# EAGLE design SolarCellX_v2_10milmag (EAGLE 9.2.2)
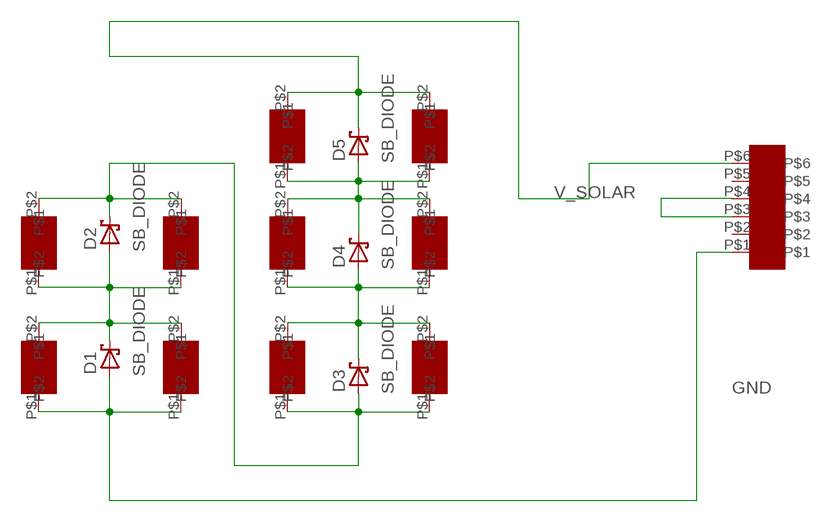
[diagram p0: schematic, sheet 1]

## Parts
1  SLMD121H04L  [SLMD121H04L]
2  SLMD121H04L  [SLMD121H04L]
11  SLMD121H04L  [SLMD121H04L]
12  SLMD121H04L  [SLMD121H04L]
13  SLMD121H04L  [SLMD121H04L]
14  SLMD121H04L  [SLMD121H04L]
21  SLMD121H04L  [SLMD121H04L]
22  SLMD121H04L  [SLMD121H04L]
23  SLMD121H04L  [SLMD121H04L]
24  SLMD121H04L  [SLMD121H04L]
D1  SB_DIODE  [SB_DIODE]
D2  SB_DIODE  [SB_DIODE]
D3  SB_DIODE  [SB_DIODE]
D4  SB_DIODE  [SB_DIODE]
D5  SB_DIODE  [SB_DIODE]
U$1  M20-8760342  [M20-8760342]

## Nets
GND: 11.P$1 12.P$1 D1.POS U$1.P$1
N$2: 11.P$2 12.P$2 13.P$1 14.P$1 D1.NEG D2.POS
N$3: 13.P$2 14.P$2 21.P$1 22.P$1 D2.NEG D3.POS
N$4: 1.P$1 2.P$1 23.P$2 24.P$2 D4.NEG D5.POS
N$5: 21.P$2 22.P$2 23.P$1 24.P$1 D3.NEG D4.POS
N$6: U$1.P$3 U$1.P$4
V_SOLAR: 1.P$2 2.P$2 D5.NEG U$1.P$6
Unconnected: U$1.P$2 U$1.P$5

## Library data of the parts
1 2 11-14 21-24 = Solar:SLMD121H04L
D1-D5 = Solar:SB_DIODE
U$1 = Solar:M20-8760342

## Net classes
1 power: width 0.254 mm

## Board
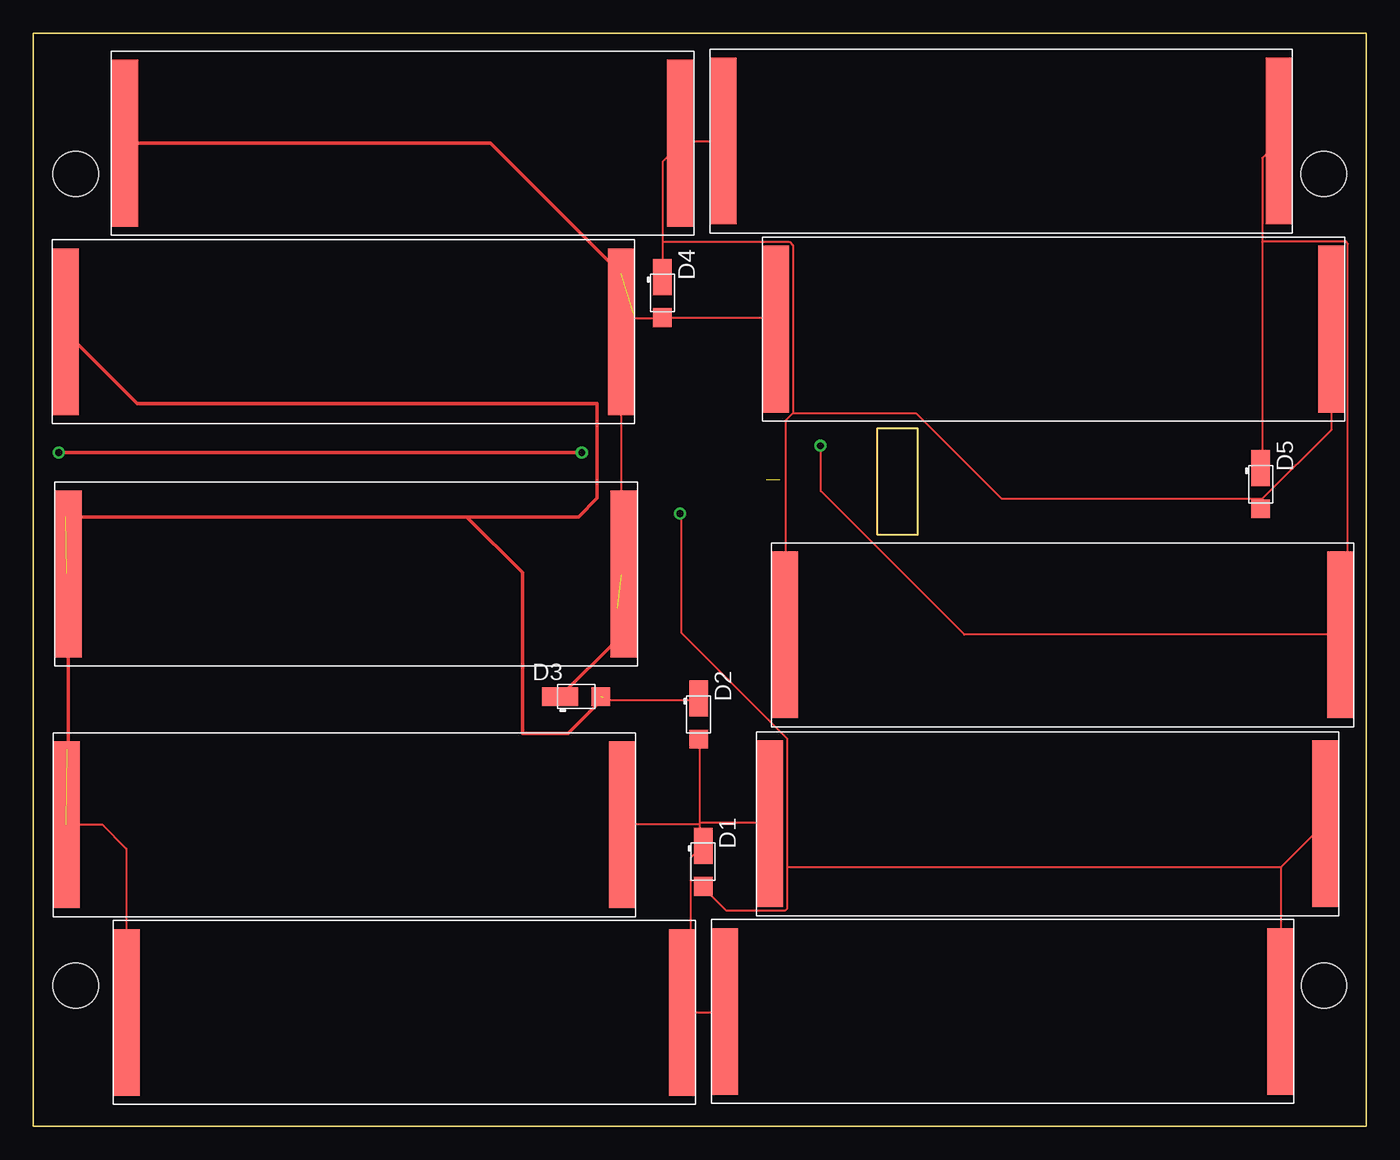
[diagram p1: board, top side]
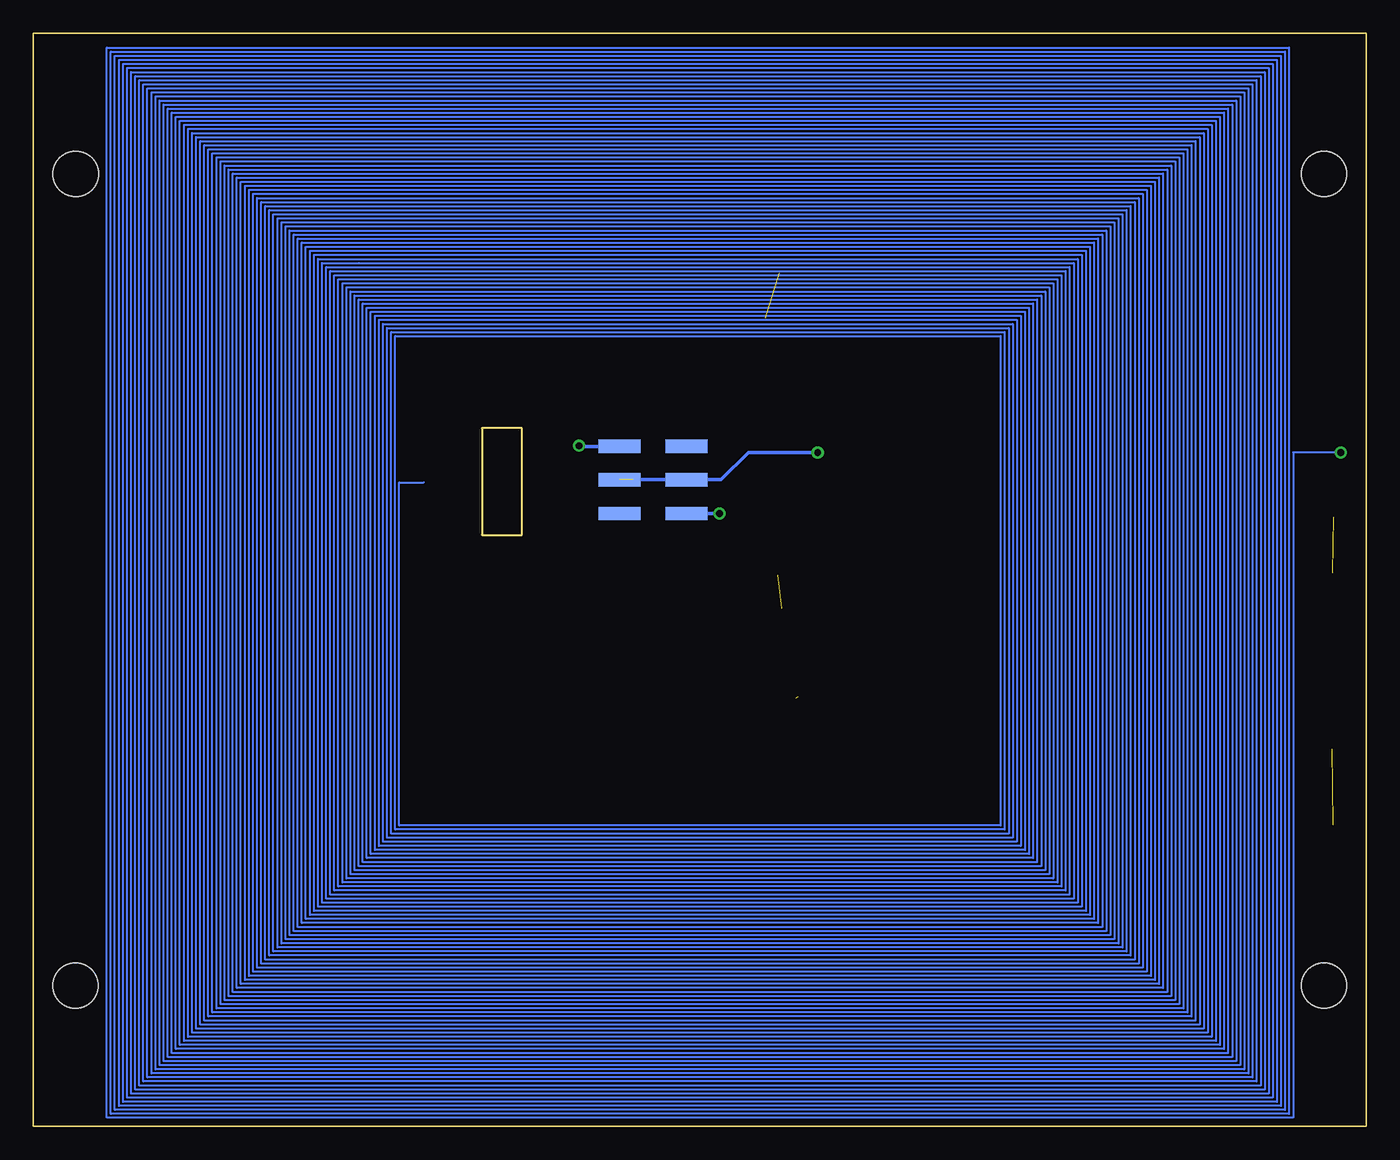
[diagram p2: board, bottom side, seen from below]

Size 100 x 82 mm. Coordinates in mm from the lower left corner, seen from the top.
Outline: 0,0 0,82 100,82 100,0 0,0
Outline: 63.35,52.37 66.35,52.37 66.35,44.37 63.35,44.37 63.35,52.37
Copper layers ([2:1+2*15+16:15]): Top 0.035559375mm / dielectric 0.17018125mm / Route2 0.01778125mm / dielectric 47mil / Route15 0.01778125mm / dielectric 0.17018125mm / Bottom 0.035559375mm
Design rules "default *": minimum track width 6mil, minimum drill 0.35mm, track to track 5mil, track to pad 6mil, pad to pad 6mil, via to via 6mil, smd to smd 6mil, copper to edge 20mil, drill to drill 6mil, minimum pad ring 10mil, minimum via ring 8mil, stop-mask expansion 4mil, vias tented up to drill 0mil, thermal gap 10mil
Holes 3.4 mm at 3.17,10.55 96.82,71.45 3.17,71.45 96.83,10.55

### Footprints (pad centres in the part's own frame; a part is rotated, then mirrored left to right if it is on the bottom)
SLMD121H04L = smd 2 x 12.5: P$1 1,6.9; P$2 42.7,6.9
SB_DIODE = smd 2.7 x 1.4: NEG -1.2,0 | smd 1.4 x 1.4: POS 1.85,0
M20-8760342 = smd 1 x 3.15: P$1 0.5,1.575; P$2 0.5,6.625; P$3 3.04,1.575; P$4 3.04,6.625; P$5 5.54,1.575; P$6 5.54,6.625

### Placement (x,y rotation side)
1  50.77,67.02 0 top
2  55.37,29.97 0 top
11  94.58,15.51 180 top
12  97.95,29.59 180 top
13  49.69,15.44 180 top
14  45.18,29.52 180 top
21  1.61,34.53 0 top
22  1.41,52.7 0 top
23  5.85,66.86 0 top
24  54.7,52.9 0 top
D1  50.26,19.85 270 top
D2  49.92,30.9 270 top
D3  40.73,32.23 0 top
D4  47.19,62.52 270 top
D5  92.08,48.17 270 top
U$1  49.4,45.47 90 bottom

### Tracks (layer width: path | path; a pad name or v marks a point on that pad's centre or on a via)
GND  (via drill 0.5)
  Top 0.152: 56.58,19.42 56.58,16.34 56.44,16.2 51.97,16.2 50.29,17.88 D1.POS | 56.58,19.42 56.58,29.06 48.62,37.02 48.62,45.96 v48.51,45.97 | 93.6,19.42 93.6,8.66 11.P$1 | 93.6,19.42 96.81,22.63 12.P$1 | 93.6,19.42 56.58,19.42
  Bottom 0.254: U$1.P$1 v48.51,45.97
N$2
  Top 0.152: 49.31,8.52 51.83,8.52 11.P$2 | 49.31,8.52 48.76,8.52 13.P$1 49.31,8.52 | 50.01,22.63 50.01,21.23 50.15,21.09 D1.NEG 50.15,20.95 49.31,20.12 49.31,8.52 | 50.01,22.63 50.01,22.77 | 50.01,22.77 50.01,28.92 D2.POS | 50.01,22.77 55.18,22.77 12.P$2 | 50.01,22.63 44.28,22.63 14.P$1
N$3  (3 unrouted)
  Top 0.152: 14.P$2 2.52,22.63 5.17,22.63 6.99,20.82 6.99,8.66 13.P$2 | D2.NEG 49.87,31.99 42.49,31.99 D3.POS | 2.52,59.51 22.P$1 | 2.52,41.49 21.P$1
  Top 0.254: 22.P$1 7.78,54.23 42.29,54.23 42.29,47.12 40.89,45.72 32.51,45.72 | 32.51,45.72 2.41,45.72 | 21.P$1 2.61,28.39 2.54,28.32 | 32.51,45.72 36.7,41.53 36.7,29.46 40.13,29.46 42.8,32.13
N$4
  Top 0.152: 92.2,47.08 92.2,46.38 D5.POS | 92.2,47.08 97.37,52.25 97.37,59.79 24.P$2 | 47.22,66.36 47.22,72.36 48.48,73.62 23.P$2 48.62,73.76 48.76,73.9 51.69,73.9 1.P$1 | 47.22,66.36 47.22,63.84 D4.NEG | 57,53.51 56.44,52.95 56.44,36.88 2.P$1 | 57,53.51 57,66.08 56.72,66.36 47.22,66.36 | 92.2,47.08 72.64,47.08 66.22,53.51 57,53.51
N$5  (2 unrouted)
  Top 0.152: 24.P$1 55.6,59.93 54.9,60.63 47.22,60.63 D4.POS 47.08,60.63 45.12,60.63 44.15,59.65 22.P$2 44.15,59.51 44.15,41.35 | 44.15,41.35 44.28,41.35 21.P$2 44.15,41.35 | 6.99,73.62 23.P$1
  Top 0.254: 23.P$1 34.32,73.76 44.07,64.01 | D3.NEG 43.81,36.52 43.81,38.86
N$6  (via drill 0.5)  (1 unrouted)
  Top 0.254: v41.15,50.55 v1.91,50.55
  Bottom 0.152: v1.91,50.55 5.49,50.55 5.49,0.65 94.49,0.65 94.49,80.92 5.79,80.92 5.79,0.91 94.18,0.91 94.18,80.62 6.1,80.62 6.1,1.22 93.88,1.22 93.88,80.31 6.4,80.31 6.4,1.52 93.57,1.52 93.57,80.01 6.71,80.01 6.71,1.83 93.27,1.83 93.27,79.7 7.01,79.7 7.01,2.13 92.96,2.13 92.96,79.4 7.32,79.4 7.32,2.44 92.66,2.44 92.66,79.1 7.62,79.1 7.62,2.74 92.35,2.74 92.35,78.79 7.92,78.79 7.92,3.05 92.05,3.05 92.05,78.49 8.23,78.49 8.23,3.35 91.75,3.35 91.75,78.18 8.53,78.18 8.53,3.66 91.44,3.66 91.44,77.88 8.84,77.88 8.84,3.96 91.14,3.96 91.14,77.57 9.14,77.57 9.14,4.27 90.83,4.27 90.83,77.27 9.45,77.27 9.45,4.57 90.53,4.57 90.53,76.96 9.75,76.96 9.75,4.88 90.22,4.88 90.22,76.66 10.06,76.66 10.06,5.18 89.92,5.18 89.92,76.35 10.36,76.35 10.36,5.49 89.61,5.49 89.61,76.05 10.67,76.05 10.67,5.79 89.31,5.79 89.31,75.74 10.97,75.74 10.97,6.1 89,6.1 89,75.44 11.28,75.44 11.28,6.4 88.7,6.4 88.7,75.13 11.58,75.13 11.58,6.71 88.39,6.71 88.39,74.83 11.89,74.83 11.89,7.01 88.09,7.01 88.09,74.52 12.19,74.52 12.19,7.32 87.78,7.32 87.78,74.22 12.5,74.22 12.5,7.62 87.48,7.62 87.48,73.91 12.8,73.91 12.8,7.92 87.17,7.92 87.17,73.61 13.11,73.61 13.11,8.23 86.87,8.23 86.87,73.3 13.41,73.3 13.41,8.53 86.56,8.53 86.56,73 13.72,73 13.72,8.84 86.26,8.84 86.26,72.69 14.02,72.69 14.02,9.14 85.95,9.14 85.95,72.39 14.33,72.39 14.33,9.45 85.65,9.45 85.65,72.08 14.63,72.08 14.63,9.75 85.34,9.75 85.34,71.78 14.94,71.78 14.94,10.06 85.04,10.06 85.04,71.48 15.24,71.48 15.24,10.36 84.73,10.36 84.73,71.17 15.54,71.17 15.54,10.67 84.43,10.67 84.43,70.87 15.85,70.87 15.85,10.97 84.12,10.97 84.12,70.56 16.15,70.56 16.15,11.28 83.82,11.28 83.82,70.26 16.46,70.26 16.46,11.58 83.52,11.58 83.52,69.95 16.76,69.95 16.76,11.89 83.21,11.89 83.21,69.65 17.07,69.65 17.07,12.19 82.91,12.19 82.91,69.34 17.37,69.34 17.37,12.5 82.6,12.5 82.6,69.04 17.68,69.04 17.68,12.8 82.3,12.8 82.3,68.73 17.98,68.73 17.98,13.11 81.99,13.11 81.99,68.43 18.29,68.43 18.29,13.41 81.69,13.41 81.69,68.12 18.59,68.12 18.59,13.72 81.38,13.72 81.38,67.82 18.9,67.82 18.9,14.02 81.08,14.02 81.08,67.51 19.2,67.51 19.2,14.33 80.77,14.33 80.77,67.21 19.51,67.21 19.51,14.63 80.47,14.63 80.47,66.9 19.81,66.9 19.81,14.94 80.16,14.94 80.16,66.6 20.12,66.6 20.12,15.24 79.86,15.24 79.86,66.29 20.42,66.29 20.42,15.54 79.55,15.54 79.55,65.99 20.73,65.99 20.73,15.85 79.25,15.85 79.25,65.68 21.03,65.68 21.03,16.15 78.94,16.15 78.94,65.38 21.34,65.38 21.34,16.46 78.64,16.46 78.64,65.08 21.64,65.08 21.64,16.76 78.33,16.76 78.33,64.77 75.59,64.77 21.95,64.77 21.95,17.07 78.03,17.07 78.03,64.47 22.25,64.47 22.25,17.37 77.72,17.37 77.72,64.16 22.55,64.16 22.55,17.68 77.42,17.68 77.42,63.86 22.86,63.86 22.86,17.98 77.11,17.98 77.11,63.55 23.16,63.55 23.16,18.29 76.81,18.29 76.81,63.25 23.47,63.25 23.47,18.59 76.5,18.59 76.5,62.94 23.77,62.94 23.77,18.9 76.2,18.9 76.2,62.64 24.08,62.64 24.08,19.2 75.89,19.2 75.89,62.33 24.38,62.33 24.38,19.51 75.59,19.51 75.59,62.03 24.69,62.03 24.69,19.81 75.29,19.81 75.29,61.72 24.99,61.72 24.99,20.12 74.98,20.12 74.98,61.42 25.3,61.42 25.3,20.42 74.68,20.42 74.68,61.11 25.6,61.11 25.6,20.73 74.37,20.73 74.37,60.81 25.91,60.81 25.91,21.03 74.07,21.03 74.07,60.5 26.21,60.5 26.21,21.34 73.76,21.34 73.76,60.2 26.52,60.2 26.52,21.64 73.46,21.64 73.46,59.89 26.82,59.89 26.82,21.95 73.15,21.95 73.15,59.59 27.13,59.59 27.13,22.25 72.85,22.25 72.85,59.28 27.43,59.28 27.43,22.55 72.54,22.55 72.54,48.31 70.71,48.31
  Bottom 0.254: 54.99,48.51 U$1.P$3 48.4,48.51 46.35,50.55 v41.15,50.55
V_SOLAR  (via drill 0.5)
  Top 0.152: 92.2,66.36 92.2,72.64 93.46,73.9 1.P$2 | 92.2,66.36 92.2,49.45 D5.NEG | v59.05,51.05 59.09,50.99 59.09,47.64 69.85,36.88 98.07,36.88 2.P$2 98.21,36.88 98.63,37.3 98.63,66.22 98.49,66.36 92.2,66.36
  Bottom 0.254: U$1.P$6 59.05,51.01 v59.05,51.05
